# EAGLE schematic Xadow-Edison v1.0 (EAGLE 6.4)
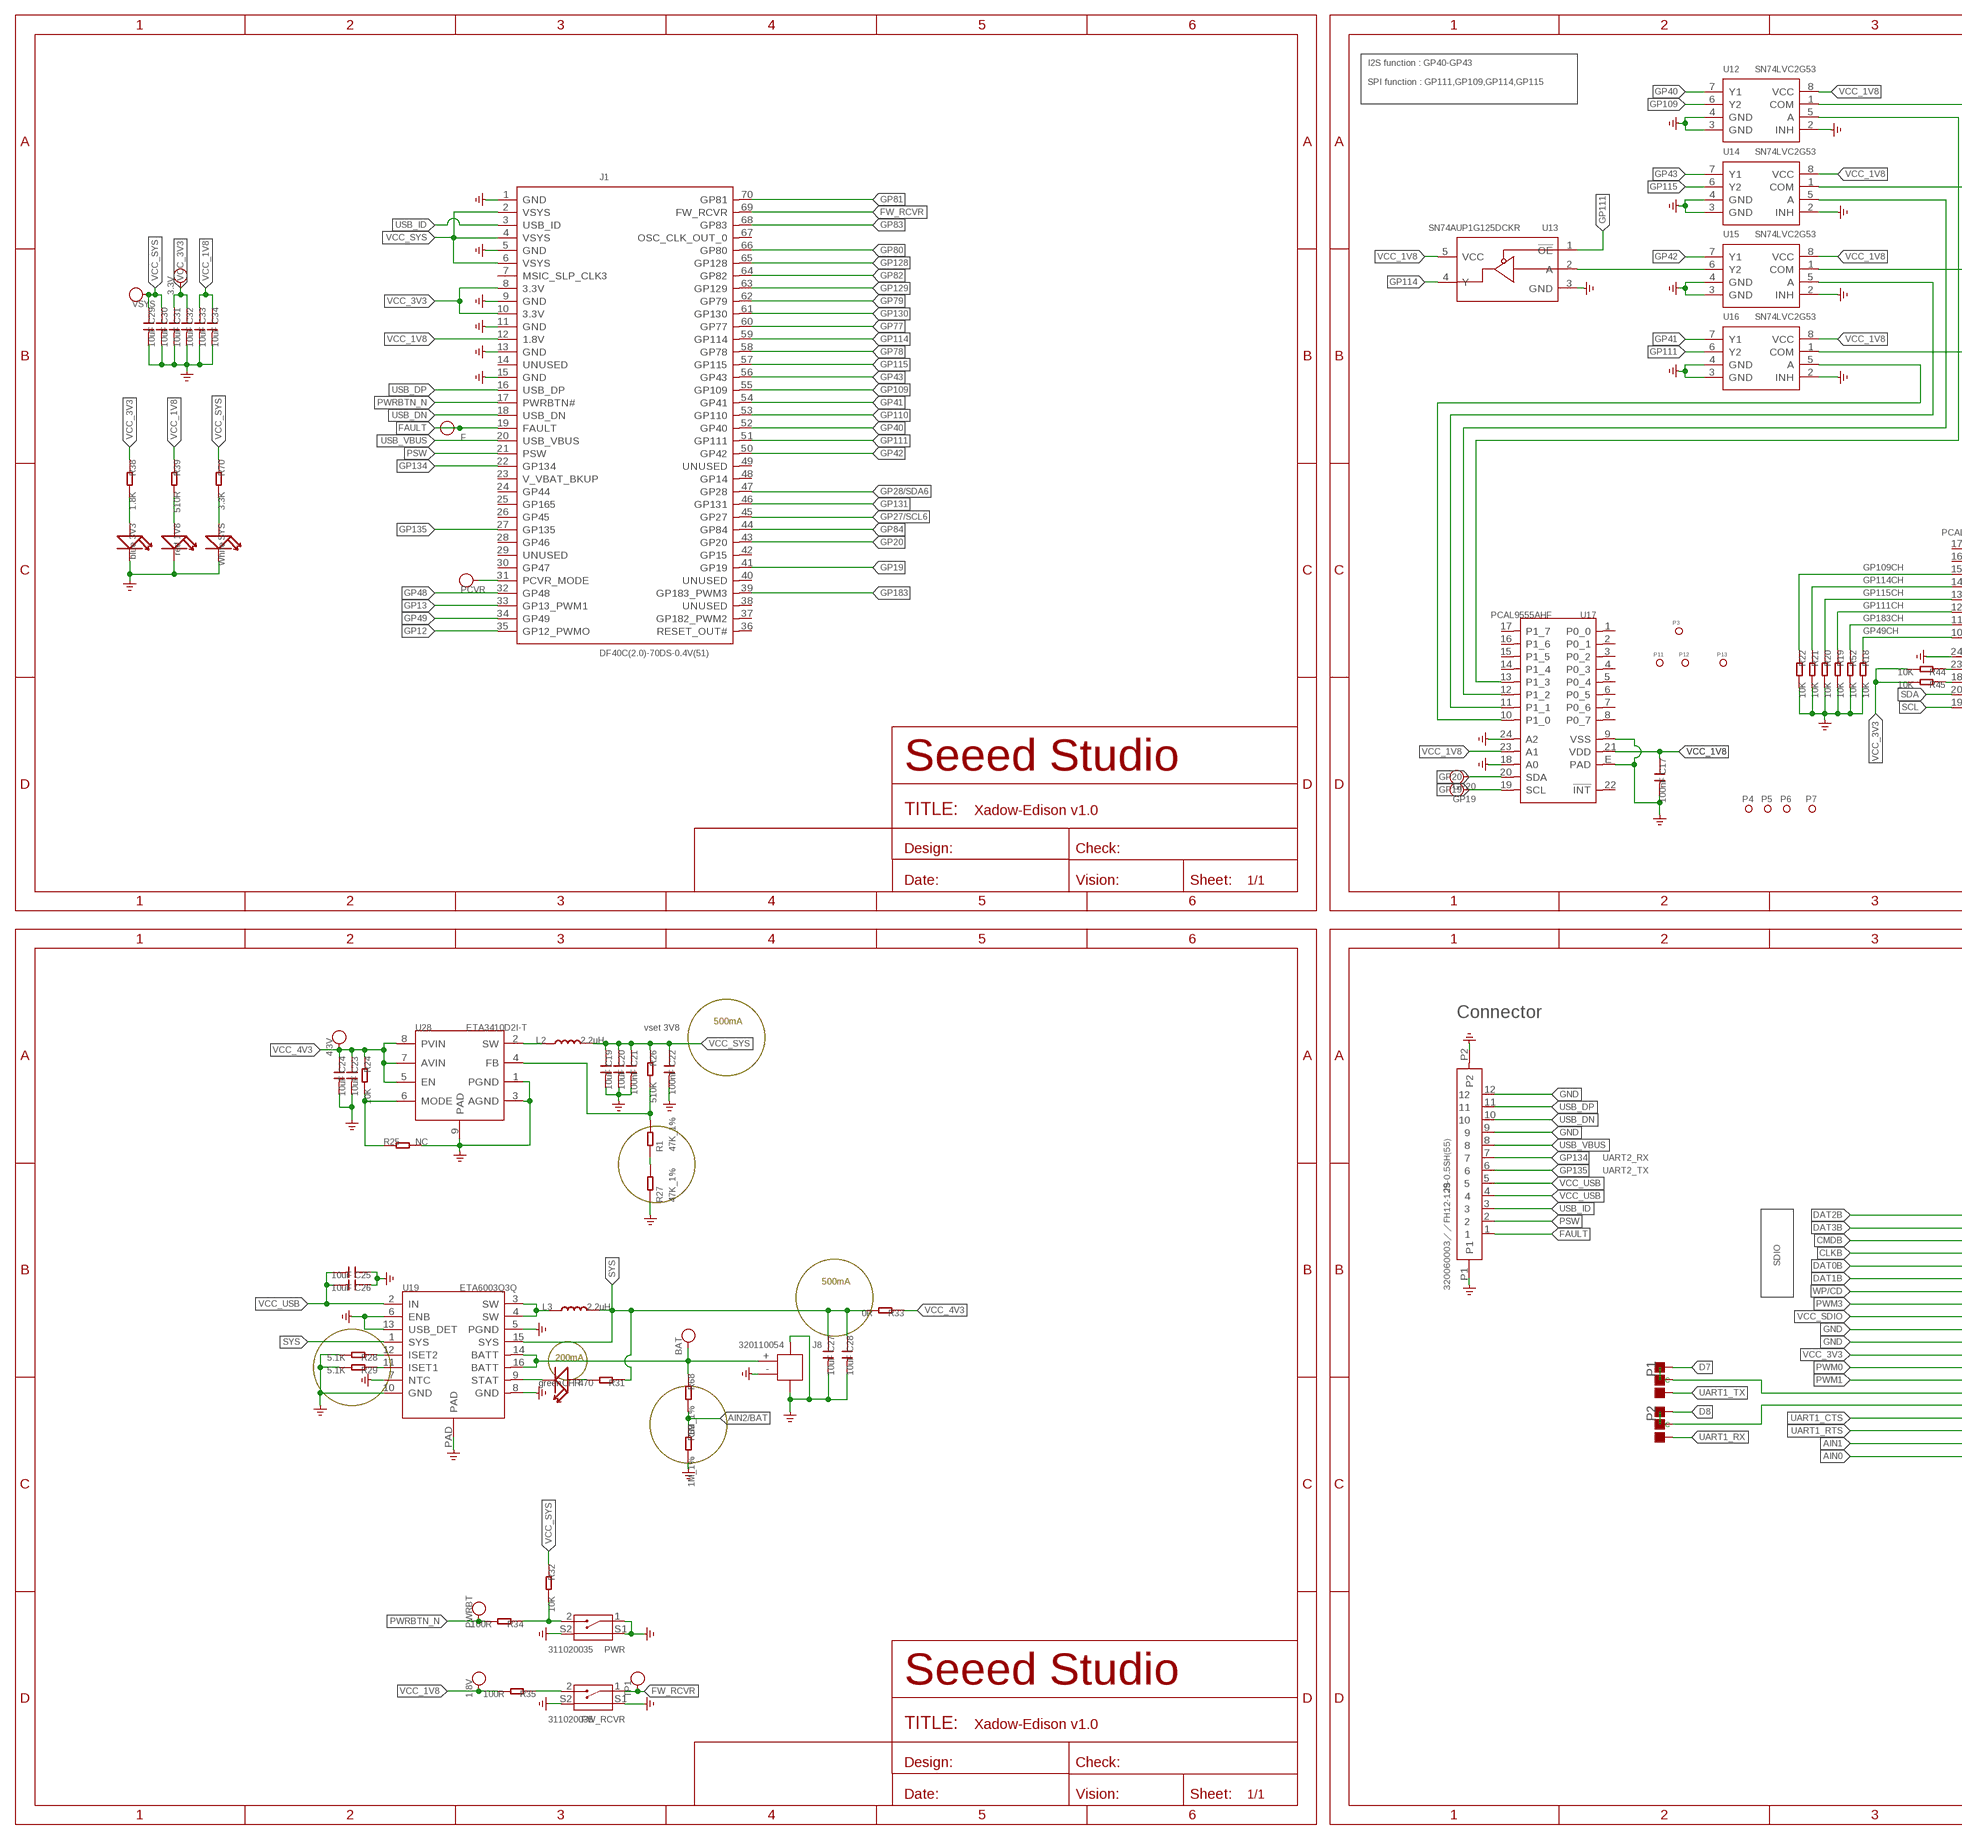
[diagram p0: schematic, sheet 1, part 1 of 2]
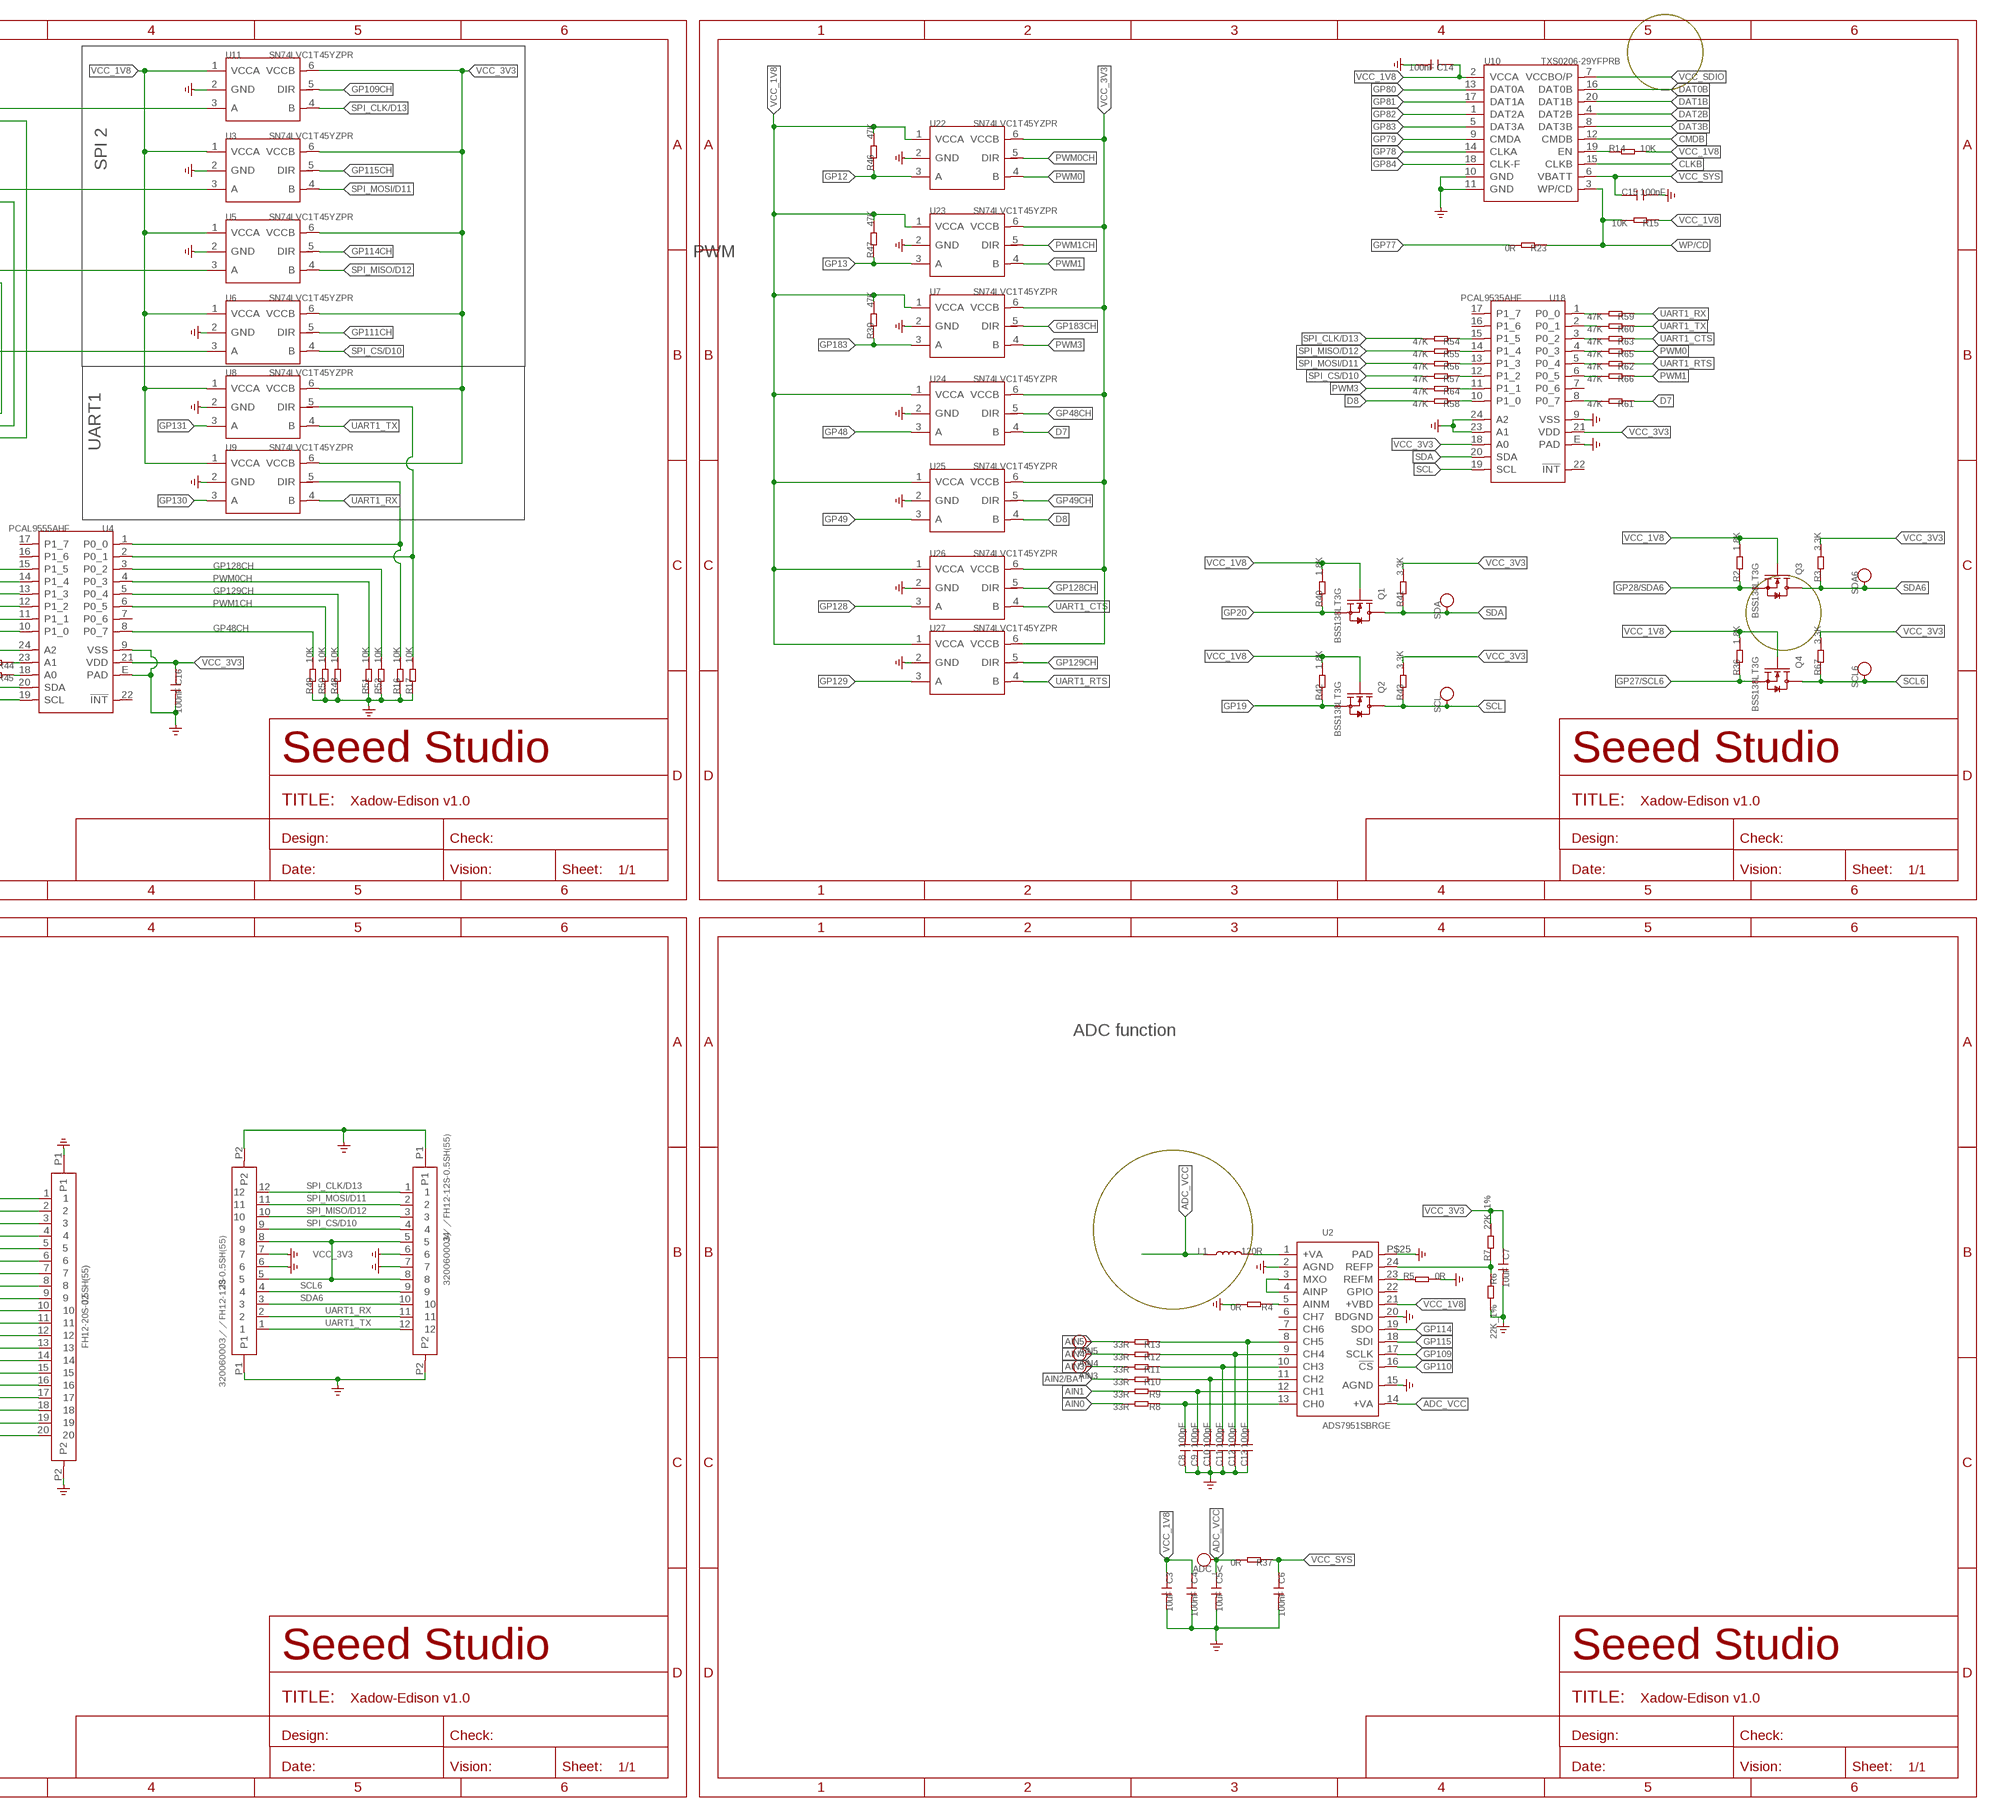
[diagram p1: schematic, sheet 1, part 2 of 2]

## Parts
1.8V  PAD-TEST-POINT'4545'  [TP-D45MIL]
1V8  red  LED'0402'  [LED-0402]
3.3V  PAD-TEST-POINT'4545'  [TP-D45MIL]
3V3  blue  LED'0402'  [LED-0402]
4.3V  PAD-TEST-POINT'4545'  [TP-D45MIL]
ADC_V  PAD-TEST-POINT'4545'  [TP-D45MIL]
AIN3  PAD-TEST-POINT'4545'  [TP-D45MIL]
AIN4  PAD-TEST-POINT'4545'  [TP-D45MIL]
AIN5  PAD-TEST-POINT'4545'  [TP-D45MIL]
BAT  PAD-TEST-POINT'4545'  [TP-D45MIL]
C3  10uF  C-0402  [C0402]
C4  100nF  C-0402  [C0402]
C5  10uF  C-0402  [C0402]
C6  100nF  C-0402  [C0402]
C7  10uF  C-0402  [C0402]
C8  100pF  C-0402  [C0402]
C9  100pF  C-0402  [C0402]
C10  100pF  C-0402  [C0402]
C11  100pF  C-0402  [C0402]
C12  100pF  C-0402  [C0402]
C13  100pF  C-0402  [C0402]
C14  100nF  C-0402  [C0402]
C15  100nF  C-0402  [C0402]
C16  100nF  C-0402  [C0402]
C17  100nF  C-0402  [C0402]
C19  10uF  C-0402  [C0402]
C20  10uF  C-0402  [C0402]
C21  100nF  C-0402  [C0402]
C22  100nF  C-0402  [C0402]
C23  10uF  C-0402  [C0402]
C24  10uF  C-0402  [C0402]
C25  10uF  C-0402  [C0402]
C26  10uF  C-0402  [C0402]
C27  10uF  C-0402  [C0402]
C28  10uF  C-0402  [C0402]
C29  10uF  C-0402  [C0402]
C30  10uF  C-0402  [C0402]
C31  10uF  C-0402  [C0402]
C32  10uF  C-0402  [C0402]
C33  10uF  C-0402  [C0402]
C34  10uF  C-0402  [C0402]
CHR  green  LED'0402'  [LED-0402]
F  PAD-TEST-POINT  [TP-D23MIL]
FW_RCVR  311020035  BUTTON-2+2P'HQ-TP-1100A'  [4P-SMD-L4.5*W3.8*H1.8MM-90D]
GP19  PAD-TEST-POINT  [TP-D23MIL]
GP20  PAD-TEST-POINT  [TP-D23MIL]
J1  DF40C(2.0)-70DS-0.4V(51)  DF40GB(3.0)-70DS-0.4V(51)  [70PIN-SMD-L16.64*W3.38*H3.12MM]
J2  FH12-20S-0.5SH(55)  FH12-20S-0.5SH(55)FH12-20S-0.5SH  [20P-0.5]
J3  320060003／／FH12-12S-0.5SH(55)  FPC052002-12LT-FH12-12S-0.5SH  [12P-0.5-NEW]
J4  320060003／／FH12-12S-0.5SH(55)  FPC052002-12LT-FH12-12S-0.5SH  [12P-0.5-NEW]
J8  320110054  JST-2P-SMD'1.0'  [2P-SMD-1.0-90D]
J9  320060003／／FH12-12S-0.5SH(55)  FPC052002-12LT-FH12-12S-0.5SH  [12P-0.5-NEW]
L1  120R  L'0805'  [L0805]
L2  2.2uH  L'0805'  [L0805]
L3  2.2uH  L'0805'  [L0805]
P1  PAD-JUMPER-3P-40*40  [3P-SMD-4.1X1.5]
P2  PAD-JUMPER-3P-40*40  [3P-SMD-4.1X1.5]
P3  DNP  PAD-MARK'ANNULAR'  [ROUND-MARK-1.0]
P4  PAD-MARK'ANNULAR'  [ROUND-MARK-1.0]
P5  PAD-MARK'ANNULAR'  [ROUND-MARK-1.0]
P6  PAD-MARK'ANNULAR'  [ROUND-MARK-1.0]
P7  PAD-MARK'ANNULAR'  [ROUND-MARK-1.0]
P11  DNP  PAD-MARK'ANNULAR'  [ROUND-MARK-1.0]
P12  √  PAD-MARK'ANNULAR'  [ROUND-MARK-1.0]
P13  √  PAD-MARK'ANNULAR'  [ROUND-MARK-1.0]
PCVR  PAD-TEST-POINT  [TP-D23MIL]
PWR  311020035  BUTTON-2+2P'HQ-TP-1100A'  [4P-SMD-L4.5*W3.8*H1.8MM-90D]
PWRBT  PAD-TEST-POINT'4545'  [TP-D45MIL]
Q1  BSS138LT3G  MOSFET-N'SI1304BDL'  [SOT-323]
Q2  BSS138LT3G  MOSFET-N'SI1304BDL'  [SOT-323]
Q3  BSS138LT3G  MOSFET-N'SI1304BDL'  [SOT-323]
Q4  BSS138LT3G  MOSFET-N'SI1304BDL'  [SOT-323]
R1  47K_1%  R-0402  [R0402]
R2  1.8K  R-0402  [R0402]
R3  3.3K  R-0402  [R0402]
R4  0R  R-0402  [R0402]
R5  0R  R-0402  [R0402]
R6  22K_1%  R-0402  [R0402]
R7  22K_1%  R-0402  [R0402]
R8  33R  R-0402  [R0402]
R9  33R  R-0402  [R0402]
R10  33R  R-0402  [R0402]
R11  33R  R-0402  [R0402]
R12  33R  R-0402  [R0402]
R13  33R  R-0402  [R0402]
R14  10K  R-0402  [R0402]
R15  10K  R-0402  [R0402]
R16  10K  R-0402  [R0402]
R17  10K  R-0402  [R0402]
R18  10K  R-0402  [R0402]
R19  10K  R-0402  [R0402]
R20  10K  R-0402  [R0402]
R21  10K  R-0402  [R0402]
R22  10K  R-0402  [R0402]
R23  0R  R-0402  [R0402]
R24  10K  R-0402  [R0402]
R25  NC  R-0402  [R0402]
R26  510K  R-0402  [R0402]
R27  47K_1%  R-0402  [R0402]
R28  5.1K  R-0402  [R0402]
R29  5.1K  R-0402  [R0402]
R30  47K  R-0402  [R0402]
R31  470  R-0402  [R0402]
R32  10K  R-0402  [R0402]
R33  0R  R-0402  [R0402]
R34  100R  R-0402  [R0402]
R35  100R  R-0402  [R0402]
R36  1.8K  R-0402  [R0402]
R37  0R  R-0402  [R0402]
R38  1.8K  R-0402  [R0402]
R39  510R  R-0402  [R0402]
R40  1.8K  R-0402  [R0402]
R41  3.3K  R-0402  [R0402]
R42  1.8K  R-0402  [R0402]
R43  3.3K  R-0402  [R0402]
R44  10K  R-0402  [R0402]
R45  10K  R-0402  [R0402]
R46  47K  R-0402  [R0402]
R47  47K  R-0402  [R0402]
R48  10K  R-0402  [R0402]
R49  10K  R-0402  [R0402]
R50  10K  R-0402  [R0402]
R51  10K  R-0402  [R0402]
R52  10K  R-0402  [R0402]
R53  10K  R-0402  [R0402]
R54  47K  R-0402  [R0402]
R55  47K  R-0402  [R0402]
R56  47K  R-0402  [R0402]
R57  47K  R-0402  [R0402]
R58  47K  R-0402  [R0402]
R59  47K  R-0402  [R0402]
R60  47K  R-0402  [R0402]
R61  47K  R-0402  [R0402]
R62  47K  R-0402  [R0402]
R63  47K  R-0402  [R0402]
R64  47K  R-0402  [R0402]
R65  47K  R-0402  [R0402]
R66  47K  R-0402  [R0402]
R67  3.3K  R-0402  [R0402]
R68  1M_1%  R-0402  [R0402]
R69  1M_1%  R-0402  [R0402]
R70  3.3K  R-0402  [R0402]
SCL  PAD-TEST-POINT  [TP-D23MIL]
SCL6  PAD-TEST-POINT  [TP-D23MIL]
SDA  PAD-TEST-POINT  [TP-D23MIL]
SDA6  PAD-TEST-POINT  [TP-D23MIL]
SYS  White  LED'0402'  [LED-0402]
TP1  PAD-TEST-POINT'4545'  [TP-D45MIL]
U2  ADS7951SBRGE  ADS7951'ADS7951'  [S-PVQFN-N24]
U3  SN74LVC1T45YZPR  [R-XBGA-N6]
U4  PCAL9555AHF  PCAL9535A  [QFN24]
U5  SN74LVC1T45YZPR  [R-XBGA-N6]
U6  SN74LVC1T45YZPR  [R-XBGA-N6]
U7  SN74LVC1T45YZPR  [R-XBGA-N6]
U8  SN74LVC1T45YZPR  [R-XBGA-N6]
U9  SN74LVC1T45YZPR  [R-XBGA-N6]
U10  TXS0206-29YFPRB  TXS0206-29  [R-XBGA-N20]
U11  SN74LVC1T45YZPR  [R-XBGA-N6]
U12  SN74LVC2G53  SN74LVC2G53'DCU'  [US-8]
U13  SN74AUP1G125DCKR  SN74AUP1G125'DCK'  [SOT-353]
U14  SN74LVC2G53  SN74LVC2G53'DCU'  [US-8]
U15  SN74LVC2G53  SN74LVC2G53'DCU'  [US-8]
U16  SN74LVC2G53  SN74LVC2G53'DCU'  [US-8]
U17  PCAL9555AHF  PCAL9535A  [QFN24]
U18  PCAL9535AHF  PCAL9535A  [QFN24]
U19  ETA6003Q3Q  ETA6003  [QFN16]
U22  SN74LVC1T45YZPR  [R-XBGA-N6]
U23  SN74LVC1T45YZPR  [R-XBGA-N6]
U24  SN74LVC1T45YZPR  [R-XBGA-N6]
U25  SN74LVC1T45YZPR  [R-XBGA-N6]
U26  SN74LVC1T45YZPR  [R-XBGA-N6]
U27  SN74LVC1T45YZPR  [R-XBGA-N6]
U28  ETA3410D2I-T  ETA3410  [DFN-8L]
VSYS  PAD-TEST-POINT'4545'  [TP-D45MIL]

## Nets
ADC_VCC: ADC_V.T C5.1 L1.1 R37.2 U2.14(+VA)
AIN0: J2.20 R8.2
AIN1: J2.19 R9.2
AIN2/BAT: R10.2 R68.2 R69.1
AIN3: AIN3.T R11.2
AIN4: AIN4.T R12.2
AIN5: AIN5.T R13.2
BAT: BAT.T J8.+ R68.1 U19.14(BATT) U19.16(BATT)
CLKB: J2.4 U10.15(CLKB)
CMDB: J2.3 U10.12(CMDB)
D7: P1.11(R) R61.1 U24.4(B)
D8: P2.11(R) R58.2 U25.4(B)
DAT0B: J2.5 U10.16(DAT0B)
DAT1B: J2.6 U10.20(DAT1B)
DAT2B: J2.1 U10.4(DAT2B)
DAT3B: J2.2 U10.8(DAT3B)
EN_SPI_CLK: U12.5(A) U17.13(P1_3)
EN_SPI_FUN: U16.5(A) U17.10(P1_0)
EN_SPI_MISO: U15.5(A) U17.11(P1_1)
EN_SPI_MOSI: U14.5(A) U17.12(P1_2)
FAULT: F.T J1.19(FAULT) J9.1
FW_RCVR: FW_RCVR.1 J1.69(FW_RCVR) TP1.T
GND: 1V8.- 3V3.- C3.2 C4.2 C5.2 C6.2 C7.2 C8.1 C9.1 C10.1 C11.1 C12.1 C13.1 C14.2 C15.2 C16.2 C17.2 C19.2 C20.2 C21.2 C22.2 C23.2 C24.2 C25.1 C26.1 C27.2 C28.2 C29.2 C30.2 C31.2 C32.2 C33.2 C34.2 FW_RCVR.S1 FW_RCVR.S2 J1.1(GND) J1.5(GND) J1.9(GND) J1.11(GND) J1.13(GND) J1.15(GND) J2.10 J2.11 J2.P1 J2.P2 J3.6 J3.7 J3.P1 J3.P2 J4.6 J4.7 J4.P1 J4.P2 J8.3 J8.4 J8.- J9.9 J9.12 J9.P1 J9.P2 PWR.1 PWR.S1 PWR.S2 R4.2 R5.2 R6.2 R16.1 R17.1 R18.2 R19.2 R20.2 R21.2 R22.2 R25.2 R27.2 R28.2 R29.2 R48.1 R49.1 R50.1 R51.1 R52.2 R53.1 R69.2 SYS.- U2.2(AGND) U2.15(AGND) U2.20(BDGND) U2.P$25(PAD) U3.2(GND) U4.9(VSS) U4.24(A2) U4.E(PAD) U5.2(GND) U6.2(GND) U7.2(GND) U8.2(GND) U9.2(GND) U10.10(GND) U10.11(GND) U11.2(GND) U12.2(INH) U12.3(GND) U12.4(GND) U13.3(GND) U14.2(INH) U14.3(GND) U14.4(GND) U15.2(INH) U15.3(GND) U15.4(GND) U16.2(INH) U16.3(GND) U16.4(GND) U17.9(VSS) U17.18(A0) U17.24(A2) U17.E(PAD) U18.9(VSS) U18.23(A1) U18.24(A2) U18.E(PAD) U19.5(PGND) U19.6(ENB) U19.7(NTC) U19.8(GND) U19.10(GND) U19.13(USB_DET) U19.PAD U22.2(GND) U23.2(GND) U24.2(GND) U25.2(GND) U26.2(GND) U27.2(GND) U28.1(PGND) U28.3(AGND) U28.9(PAD) ; supply symbol labelled GND_POWER
GP12: J1.35(GP12_PWMO) R46.1 U22.3(A)
GP13: J1.33(GP13_PWM1) R47.1 U23.3(A)
GP19: GP19.T J1.41(GP19) Q2.2(S) R42.1 U17.19(SCL)
GP20: GP20.T J1.43(GP20) Q1.2(S) R40.1 U17.20(SDA)
GP27/SCL6: J1.45(GP27) Q4.2(S) R36.1
GP28/SDA6: J1.47(GP28) Q3.2(S) R2.1
GP40: J1.52(GP40) U12.7(Y1)
GP41: J1.54(GP41) U16.7(Y1)
GP42: J1.50(GP42) U15.7(Y1)
GP43: J1.56(GP43) U14.7(Y1)
GP48: J1.32(GP48) U24.3(A)
GP48CH: R49.2 U4.8(P0_7) U24.5(DIR)
GP49: J1.34(GP49) U25.3(A)
GP49CH: R18.1 U4.10(P1_0) U25.5(DIR)
GP77: J1.60(GP77) R23.2
GP78: J1.58(GP78) U10.14(CLKA)
GP79: J1.62(GP79) U10.9(CMDA)
GP80: J1.66(GP80) U10.13(DAT0A)
GP81: J1.70(GP81) U10.17(DAT1A)
GP82: J1.64(GP82) U10.1(DAT2A)
GP83: J1.68(GP83) U10.5(DAT3A)
GP84: J1.44(GP84) U10.18(CLK-F)
GP109: J1.55(GP109) U2.17(SCLK) U12.6(Y2)
GP109CH: R22.1 U4.15(P1_5) U11.5(DIR)
GP110: J1.53(GP110) U2.16(!CS!)
GP111: J1.51(GP111) U13.1(!OE) U16.6(Y2)
GP111CH: R19.1 U4.12(P1_2) U6.5(DIR)
GP114: J1.59(GP114) U2.19(SDO) U13.4(Y)
GP114CH: R21.1 U4.14(P1_4) U5.5(DIR)
GP115: J1.57(GP115) U2.18(SDI) U14.6(Y2)
GP115CH: R20.1 U3.5(DIR) U4.13(P1_3)
GP128: J1.65(GP128) U26.3(A)
GP128CH: R53.2 U4.3(P0_2) U26.5(DIR)
GP129: J1.63(GP129) U27.3(A)
GP129CH: R48.2 U4.5(P0_4) U27.5(DIR)
GP130: J1.61(GP130) U9.3(A)
GP130CH: R16.2 U4.1(P0_0) U9.5(DIR)
GP131: J1.46(GP131) U8.3(A)
GP131CH: R17.2 U4.2(P0_1) U8.5(DIR)
GP134: J1.22(GP134) J9.7
GP135: J1.27(GP135) J9.6
GP183: J1.39(GP183_PWM3) R30.1 U7.3(A)
GP183CH: R52.1 U4.11(P1_1) U7.5(DIR)
N$1: R1.2 R27.1
N$2: R70.2 SYS.+
N$3: J1.31(PCVR_MODE) PCVR.T
N$4: R24.2 R25.1 U28.6(MODE)
N$5: CHR.+ R31.2
N$6: U11.3(A) U12.1(COM)
N$7: CHR.- U19.9(STAT)
N$8: L1.2 U2.1(+VA)
N$9: R4.1 U2.5(AINM)
N$10: U2.3(MXO) U2.4(AINP)
N$11: L2.1 U28.2(SW)
N$12: R5.1 U2.23(REFM)
N$13: R44.1 U4.23(A1)
N$14: R6.1 R7.1 U2.24(REFP)
N$15: C8.2 R8.1 U2.13(CH0)
N$16: C12.2 R12.1 U2.9(CH4)
N$17: C13.2 R13.1 U2.8(CH5)
N$18: C9.2 R9.1 U2.12(CH1)
N$19: C10.2 R10.1 U2.11(CH2)
N$20: C11.2 R11.1 U2.10(CH3)
N$21: J2.15 P1.MM(C)
N$23: U3.3(A) U14.1(COM)
N$24: J2.16 P2.MM(C)
N$27: R59.2 U18.1(P0_0)
N$28: R58.1 U18.10(P1_0)
N$29: R54.1 U18.15(P1_5)
N$30: R57.1 U18.12(P1_2)
N$31: R56.1 U18.13(P1_3)
N$32: R55.1 U18.14(P1_4)
N$33: R60.2 U18.2(P0_1)
N$34: R61.2 U18.8(P0_7)
N$35: R14.1 U10.19(EN)
N$36: R64.1 U18.11(P1_1)
N$37: R62.2 U18.5(P0_4)
N$38: R63.2 U18.3(P0_2)
N$39: R65.2 U18.4(P0_3)
N$40: R66.2 U18.6(P0_5)
N$43: R45.1 U4.18(A0)
N$44: U5.3(A) U15.1(COM)
N$45: R1.1 R26.2 U28.4(FB)
N$46: FW_RCVR.2 R35.1
N$47: L3.1 U19.3(SW) U19.4(SW)
N$48: U6.3(A) U16.1(COM)
N$50: 3V3.+ R38.2
N$51: 1V8.+ R39.2
N$53: R28.1 U19.12(ISET2)
N$58: R29.1 U19.11(ISET1)
N$76: PWR.2 R32.2 R34.1
N$78: U13.2(A) U15.6(Y2)
PSW: J1.21(PSW) J9.2
PWM0: J2.13 R65.1 U22.4(B)
PWM0CH: R51.2 U4.4(P0_3) U22.5(DIR)
PWM1: J2.14 R66.1 U23.4(B)
PWM1CH: R50.2 U4.6(P0_5) U23.5(DIR)
PWM3: J2.8 R64.2 U7.4(B)
PWRBTN_N: J1.17(PWRBTN#) PWRBT.T R34.2
SCL: Q2.3(D) R43.1 SCL.T U4.19(SCL) U18.19(SCL)
SCL6: J3.4 J4.9 Q4.3(D) R67.1 SCL6.T
SDA: Q1.3(D) R41.1 SDA.T U4.20(SDA) U18.20(SDA)
SDA6: J3.3 J4.10 Q3.3(D) R3.1 SDA6.T
SPI_CLK/D13: J3.12 J4.1 R54.2 U11.4(B)
SPI_CS/D10: J3.9 J4.4 R57.2 U6.4(B)
SPI_MISO/D12: J3.10 J4.3 R55.2 U5.4(B)
SPI_MOSI/D11: J3.11 J4.2 R56.2 U3.4(B)
SYS: C27.1 C28.1 L3.2 R31.1 R33.2 U19.1(SYS) U19.15(SYS)
UART1_CTS: J2.17 R63.1 U26.4(B)
UART1_RTS: J2.18 R62.1 U27.4(B)
UART1_RX: J3.2 J4.11 P2.00(L) R59.1 U9.4(B)
UART1_TX: J3.1 J4.12 P1.00(L) R60.1 U8.4(B)
USB_DN: J1.18(USB_DN) J9.10
USB_DP: J1.16(USB_DP) J9.11
USB_ID: J1.3(USB_ID) J9.3
USB_VBUS: J1.20(USB_VBUS) J9.8
VCC_1V8: 1.8V.T C3.1 C4.1 C14.1 C17.1 C33.1 C34.1 J1.12(1.8V) Q1.1(G) Q2.1(G) Q3.1(G) Q4.1(G) R2.2 R14.2 R15.1 R30.2 R35.2 R36.2 R39.1 R40.2 R42.2 R46.2 R47.2 U2.21(+VBD) U3.1(VCCA) U5.1(VCCA) U6.1(VCCA) U7.1(VCCA) U8.1(VCCA) U9.1(VCCA) U10.2(VCCA) U11.1(VCCA) U12.8(VCC) U13.5(VCC) U14.8(VCC) U15.8(VCC) U16.8(VCC) U17.21(VDD) U17.23(A1) U22.1(VCCA) U23.1(VCCA) U24.1(VCCA) U25.1(VCCA) U26.1(VCCA) U27.1(VCCA)
VCC_3V3: 3.3V.T C7.1 C16.1 C31.1 C32.1 J1.8(3.3V) J1.10(3.3V) J2.12 J3.5 J3.8 J4.5 J4.8 R3.2 R7.2 R38.1 R41.2 R43.2 R44.2 R45.2 R67.2 U3.6(VCCB) U4.21(VDD) U5.6(VCCB) U6.6(VCCB) U7.6(VCCB) U8.6(VCCB) U9.6(VCCB) U11.6(VCCB) U18.18(A0) U18.21(VDD) U22.6(VCCB) U23.6(VCCB) U24.6(VCCB) U25.6(VCCB) U26.6(VCCB) U27.6(VCCB)
VCC_4V3: 4.3V.T C23.1 C24.1 R24.1 R33.1 U28.5(EN) U28.7(AVIN) U28.8(PVIN)
VCC_SDIO: J2.9 U10.7(VCCBO/P)
VCC_SYS: C6.1 C15.1 C19.1 C20.1 C21.1 C22.1 C29.1 C30.1 J1.2(VSYS) J1.4(VSYS) J1.6(VSYS) L2.2 R26.1 R32.1 R37.1 R70.1 U10.6(VBATT) VSYS.T
VCC_USB: C25.2 C26.2 J9.4 J9.5 U19.2(IN)
WP/CD: J2.7 R15.2 R23.1 U10.3(WP/CD)
Unconnected: J1.7(MSIC_SLP_CLK3) J1.14(UNUSED) J1.23(V_VBAT_BKUP) J1.24(GP44) J1.25(GP165) J1.26(GP45) J1.28(GP46) J1.29(UNUSED) J1.30(GP47) J1.36(RESET_OUT#) J1.37(GP182_PWM2) J1.38(UNUSED) J1.40(UNUSED) J1.42(GP15) J1.48(GP14) J1.49(UNUSED) J1.67(OSC_CLK_OUT_0) U2.6(CH7) U2.7(CH6) U2.22(GPIO) U4.7(P0_6) U4.16(P1_6) U4.17(P1_7) U4.22(!INT!) U17.1(P0_0) U17.2(P0_1) U17.3(P0_2) U17.4(P0_3) U17.5(P0_4) U17.6(P0_5) U17.7(P0_6) U17.8(P0_7) U17.14(P1_4) U17.15(P1_5) U17.16(P1_6) U17.17(P1_7) U17.22(!INT!) U18.7(P0_6) U18.16(P1_6) U18.17(P1_7) U18.22(!INT!)

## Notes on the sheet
- I2S function : GP40-GP43
- SPI function : GP111,GP109,GP114,GP115
- SPI 2
- PWM
- UART1
- Connector
- 500mA
- vset 3V8
- ADC function
- UART2_RX
- UART2_TX
- SDIO
- 500mA
- 200mA

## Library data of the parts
1.8V 3.3V 4.3V ADC_V AIN3-AIN5 BAT PWRBT TP1 VSYS = Discrete-new:PAD-TEST-POINT; PARTNO: DNP
1V8 3V3 CHR SYS = Discrete:LED*
C3-C17 C19-C34 = Discrete:C*: Ceramic Capacitors
F GP19 GP20 PCVR SCL SCL6 SDA SDA6 = Discrete-new:PAD-TEST-POINT
FW_RCVR PWR = Discrete-new:BUTTON-2+2P: 4P-SMD-L4.5*W3.8*H1.8MM-90D:311020035;4P-SMD-L7.0*W3.5*H3.5MM-90D:311020023
J1 = template:DF40GB(3.0)-70DS-0.4V(51): Edison 70-pin Interface Connector
J2 = template:FH12-20S-0.5SH(55)
J3 J4 J9 = template:FPC052002-12LT
J8 = Connector-new:JST-2P-SMD: 2P-SMD-1.0-90D:320110054;2P-SMD-2.0-90D:320110026
L1-L3 = Discrete:L*
P1 P2 = Discrete:PAD-JUMPER-3P; PARTNO: DNP
P3 P11-P13 = Discrete:PAD-MARK; PARTNO: DNP
P4-P7 = Discrete-new:PAD-MARK; PARTNO: DNP
Q1-Q4 = Discrete-new:MOSFET-N: IRLL014: http://www.vishay.com/docs/91319/sihll014.pdf
R1-R70 = Discrete:R*
U2 = template:ADS7951: 12/10/8-Bit,1MSPS,16/12/8/4-Channel,Single-Ended,MicroPower,Serial Interface ADCs
U3 U5-U9 U11 U22-U27 = template:SN74LVC1T45YZPR: SINGLE-BIT DUAL-SUPPLY BUS TRANSCEIVER WITH CONFIGURABLE VOLTAGE TRANSLATION AND 3-STATE OUTPUTS
U4 U17 U18 = template:PCAL9535A: Low-voltage 16-bit I2C-bus I/O port with interrupt and Agile I/O
U10 = template:TXS0206-29: MMC,SD CARD,Memory Stick TM VOLTAGE-TRANSLATION TRANSCEIVER AND LDO VOLTAGE REGULATOR WITH ESD PROTECTION AND EMI FILTERING
U12 U14-U16 = template:SN74LVC2G53: SN74LVC2G53 Single-Pole Double-Throw (SPDT) Analog Switch 2:1 Analog Multiplexer/Demultiplexer
U13 = template:SN74AUP1G125: LOW-POWER SINGLE BUS BUFFER GATE WITH 3-STATE OUTPUT
U19 = template:ETA6003: 2.5A,3MHZ Switching Charger with Dynamic Power Path Management
U28 = template:ETA3410: 3MHZ 2A High Step-Down Converter in DFN2x2-8L Package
